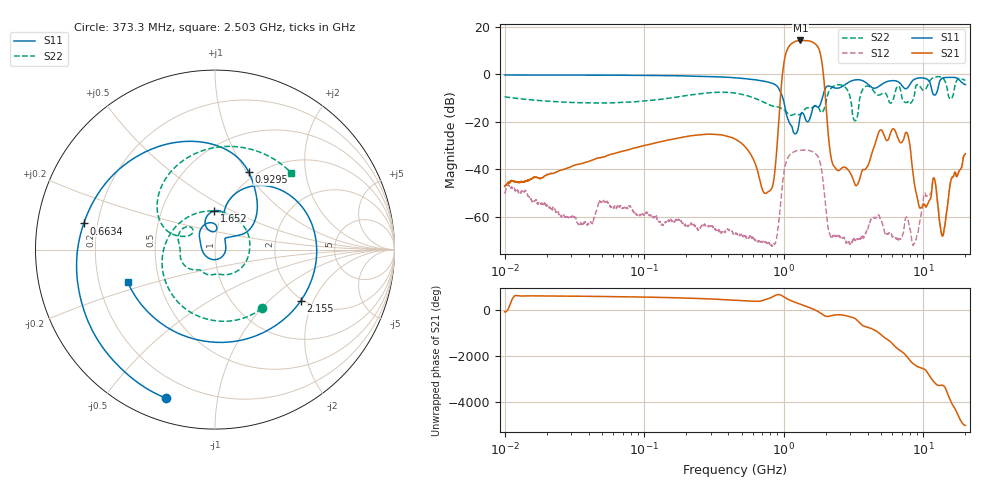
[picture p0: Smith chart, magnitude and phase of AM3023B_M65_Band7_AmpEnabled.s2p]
!Agilent Technologies,E8364B,MY43040894,A.07.50.67
!Agilent E8364B: A.07.50.67
!Date: Tuesday, October 27, 2020 10:53:58
!Correction: S11(Full 2 Port(1,2))
!S21(Full 2 Port(1,2))
!S12(Full 2 Port(1,2))
!S22(Full 2 Port(1,2))
!S2P File: Measurements: S11, S21, S12, S22:Log Frequency Sweep
# Hz S  dB  R 50
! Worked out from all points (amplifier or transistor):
!   3201 points, 10 MHz to 20 GHz, reference 50 ohm
!   highest |S21| = 14.3 dB at 1.315 GHz (marker M1)
!   |S21| within 3 dB of that: 1.077 GHz to 1.766 GHz (689.5 MHz wide, 48.5 % of centre)
!   unconditionally stable (mu >= 1): start of sweep to end of sweep
!   at 35.47 MHz: K = 4156.35, MAG = -26.3 dB, |S12| = -63.4 dB
!   at 447.2 MHz: K = 6308.02, MAG = -21.1 dB, |S12| = -67.1 dB
!   at 20 GHz: K = 335.45, MAG = -28.0 dB, |S12| = -34.0 dB
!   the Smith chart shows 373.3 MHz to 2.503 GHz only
!   S11 on the Smith chart (normalised r, x): 373.3 MHz: 0.10, -0.72; 663.4 MHz: 0.15, +0.10; 929.5 MHz: 0.92, +1.02; 1.652 GHz: 0.90, +0.41; 2.155 GHz: 1.94, -1.61; 2.503 GHz: 0.33, -0.16
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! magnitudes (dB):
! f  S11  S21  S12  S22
! 10 MHz  -0.3  -47.3  -50.2  -9.5
! 35.55 MHz  -0.4  -37.6  -63.2  -12.0
! 126.1 MHz  -0.5  -28.7  -61.6  -10.7
! 373.3 MHz  -1.2  -25.8  -66.3  -7.6
! 447.2 MHz  -1.5  -27.3  -67.1  -7.9
! 663.4 MHz  -2.5  -42.9  -70.7  -10.8
! 821.5 MHz  -3.7  -48.0  -72.1  -13.3
! 929.5 MHz  -6.5  -16.0  -60.1  -14.0
! 1.042 GHz  -16.7  9.3  -36.9  -15.8
! 1.315 GHz  -17.5  14.3  -32.0  -16.8
! 1.59 GHz  -15.6  13.7  -32.5  -14.1
! 1.652 GHz  -13.3  13.2  -33.0  -13.6
! 1.873 GHz  -10.7  5.3  -40.9  -16.1
! 2.155 GHz  -5.1  -33.2  -68.2  -6.2
! 2.503 GHz  -5.7  -40.5  -68.2  -4.4
! 3.235 GHz  -2.4  -46.5  -69.9  -19.6
! 5.639 GHz  -2.9  -27.2  -67.1  -11.0
! 7.661 GHz  -5.8  -24.9  -61.0  -11.7
! 8.627 GHz  -2.1  -46.3  -71.2  -8.7
! 11.92 GHz  -8.7  -43.8  -43.6  -1.3
! 13.68 GHz  -1.6  -68.2  -68.6  -1.4
! 20 GHz  -4.3  -33.5  -34.0  -2.6
